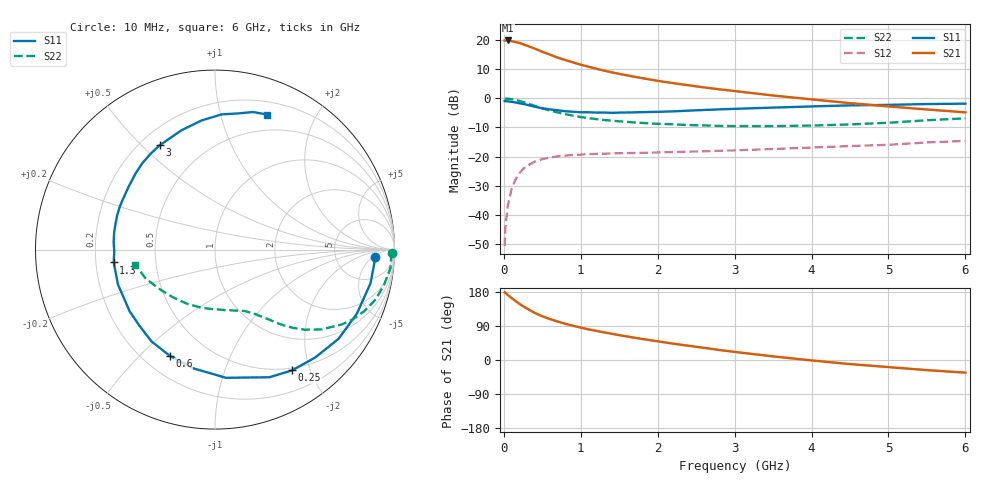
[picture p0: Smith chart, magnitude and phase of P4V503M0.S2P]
! SIEMENS Small Signal Semiconductors
! BFP182
! Si NPN RF Bipolar Junction Transistor in SOT143
! VCE = 0.5 V  IC = 3 mA
! Common Emitter S-Parameters:  March  1996
# GHz  S  MA  R  50
!  f  S11  S21  S12  S22
! GHz  MAG  ANG  MAG  ANG  MAG  ANG  MAG  ANG
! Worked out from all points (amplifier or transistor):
!   36 points, 10 MHz to 6 GHz, reference 50 ohm
!   highest |S21| = 19.8 dB at 50 MHz (marker M1)
!   |S21| within 3 dB of that: start of sweep to 420 MHz
!   unconditionally stable (mu >= 1): 1.687 GHz to end of sweep
!   at 250 MHz: K = 0.18, MSG = 21.4 dB, |S12| = -24.3 dB
!   at 1.4 GHz: K = 0.87, MSG = 13.9 dB, |S12| = -19.0 dB
!   at 6 GHz: K = 1.23, MAG = 2.0 dB, |S12| = -14.6 dB
!   S11 on the Smith chart (normalised r, x): 10 MHz: 15, -6; 250 MHz: 0.47, -1.73; 600 MHz: 0.31, -0.62; 1.3 GHz: 0.28, -0.06; 3 GHz: 0.28, +0.57; 6 GHz: 0.33, +1.41
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0.01  0.89 -2.5  9.771 178.7  0.0029 82.5  0.989 -1.1
0.02  0.8909 -4.9  9.77 177.3  0.0059 89.4  0.9827 -2.4
0.05  0.8866 -12.2  9.797 171.8  0.014 84.4  0.9831 -6.0
0.1  0.8674 -24.2  9.528 163.8  0.0275 75.3  0.9621 -11.8
0.15  0.8493 -35.8  9.209 156.0  0.0402 69.8  0.9372 -17.2
0.2  0.8204 -47.1  8.916 148.4  0.0512 63.9  0.9006 -22.3
0.25  0.7986 -57.4  8.414 141.7  0.0609 58.4  0.8602 -26.9
0.3  0.7727 -67.0  7.98 136.0  0.0693 53.9  0.8211 -30.5
0.4  0.7169 -85.1  7.115 124.4  0.0815 46.0  0.7423 -36.8
0.5  0.6721 -100.5  6.263 115.3  0.0902 39.5  0.671 -41.7
0.6  0.6427 -113.2  5.595 108.0  0.0965 34.6  0.6153 -45.1
0.7  0.6219 -124.7  4.974 101.4  0.1006 30.8  0.5701 -47.8
0.8  0.5974 -134.9  4.52 95.5  0.1038 27.7  0.5334 -49.9
1.1  0.5745 -160.2  3.481 80.8  0.11 21.5  0.4554 -55.1
1.3  0.5689 -172.8  2.983 73.0  0.112 18.7  0.4239 -57.9
1.7  0.5729 165.1  2.332 58.8  0.115 15.6  0.3833 -63.6
2.2  0.5952 144.0  1.815 43.2  0.1194 13.9  0.3574 -72.2
3  0.6578 118.0  1.328 21.4  0.1274 12.2  0.333 -90.3
3.5  0.6906 105.7  1.114 9.5  0.1348 11.3  0.3327 -103.3
4.5  0.7546 87.1  0.825 -10.8  0.1512 8.7  0.3553 -132.0
5.5  0.795 74.6  0.642 -26.7  0.1745 5.5  0.4193 -157.6
6  0.8071 68.8  0.572 -33.4  0.1852 2.2  0.4522 -169.4
